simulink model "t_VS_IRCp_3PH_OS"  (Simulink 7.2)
settings: Solver=ode3  StartTime=0.0  StopTime=0.02  FixedStep=1e-5  RelTol=1e-3

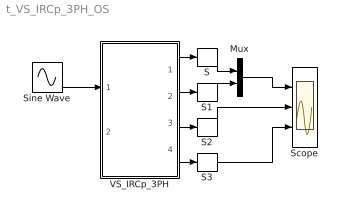
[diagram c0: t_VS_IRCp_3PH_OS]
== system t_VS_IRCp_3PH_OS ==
  Mux : Mux  Inputs=2
  S{,1..3} (4 alike) : Selector  InputPortWidth=3  IndexOptions=Index vector (dialog)  Indices=[1 ]  OutputSizes=1
  Scope : Scope  NumInputPorts=3
  Sine Wave : Sin  Amplitude=230*sqrt(2)  Frequency=1000*pi  Phase="[0  -2*pi/3  -4*pi/3]"  SampleTime=0
  VS_IRCp_3PH : Subsystem  mask(VS_IRCp_3PH_OS){R=1, C=100e-6, RCs=1}
      mask prompts: R "Load Resistance"; C "Load Capacitance"; RCs "Cap Series Res"
      mask help: Open source VS_IRCp_3PH_OS Input Vector: u[0]= Vs, Source Voltage u[1]= IL, Load Current Output Vector: y[0]=IC, Capacitor current y[1]=VC, Capacitor Voltage y[2]=IR, current of Load Resistance y[3]=VRs, Voltage on series Resistance Parameter Vector: p[0]=R1 p[1]=C p[2]=Rs
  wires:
  Sine Wave/1 -> VS_IRCp_3PH/1(V123)
  VS_IRCp_3PH/1(iC123) -> S/1
  VS_IRCp_3PH/2(vC123) -> S1/1
  Mux/1 -> Scope/1
  VS_IRCp_3PH/3(vR123) -> S2/1
  VS_IRCp_3PH/4(vRS123) -> S3/1
  S/1 -> Mux/1
  S1/1 -> Mux/2
  S2/1 -> Scope/2
  S3/1 -> Scope/3

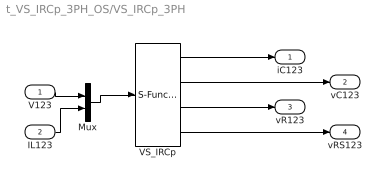
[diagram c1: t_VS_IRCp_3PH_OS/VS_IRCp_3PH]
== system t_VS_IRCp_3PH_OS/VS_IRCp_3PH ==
  V123 : Inport
  IL123 : Inport  Port=2
  Mux : Mux  Inputs=2
  VS_IRCp : S-Function  FunctionName=s_VS_IRCp_3PH_OS  Parameters=[R,C, RCs]  EnableBusSupport=off
  iC123 : Outport
  vC123 : Outport  Port=2
  vR123 : Outport  Port=3
  vRS123 : Outport  Port=4
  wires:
  Mux/1 -> VS_IRCp/1
  IL123/1 -> Mux/2
  V123/1 -> Mux/1
  VS_IRCp/1 -> iC123/1
  VS_IRCp/2 -> vC123/1
  VS_IRCp/3 -> vR123/1
  VS_IRCp/4 -> vRS123/1
